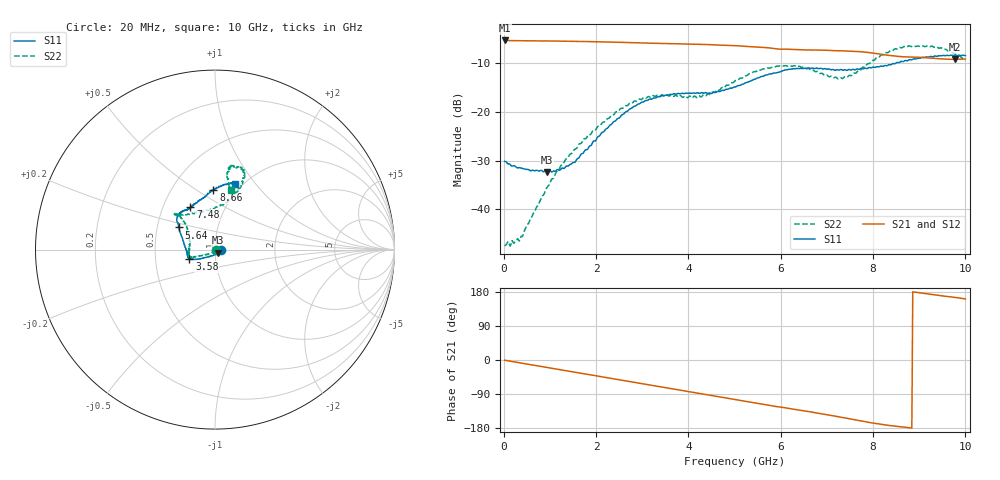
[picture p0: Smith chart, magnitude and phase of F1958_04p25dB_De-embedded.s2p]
! Integrated Device Technology
! Corporate Headquarters
! 6024 Silver Creek Valley Road
! San Jose, CA 95138  USA
! Phone:  1-408-284-8200
! Toll Free:  1-800-223-1366
! Webpage:  http://www.idt.com/
! Timing and RF Division
! 515 Groton Road, Suite 102
! Westford, MA 01886-6024
! Device:  F1958
! Description: 7-bit 0.25 dB Digital Step Attenuator
! Frequency:  0.001 -  6.000 GHz
! Package:  4x4 mm Thin QFN Plastic Package: 24 pin
! Ports:  2 RF, 12 DC
!  Pin  1  = D0
!  Pin  2  = VDD
!  Pin  3  = VMODE
!  Pin  4  = GND
!  Pin  5  = RF1  =  Port 1
!  Pin  6  = GND
!  Pin  7  = GND
!  Pin  8  = GND
!  Pin  9  = GND
!  Pin 10  = GND
!  Pin 11  = GND
!  Pin 12  = GND
!  Pin 13  = GND
!  Pin 14  = RF2  =  Port 2
!  Pin 15  = GND
!  Pin 16  = LE
!  Pin 17  = CLK
!  Pin 18  = DATA
!  Pin 19  = D6
!  Pin 20  = D5
!  Pin 21  = D4
!  Pin 22  = D3
!  Pin 23  = D2
!  Pin 24  = D1
! State:  17
! Atten State:  4.25 dB
! Voltage:  +3.30 Volts
! Current:  0.258 mA
! Data:  The device was measured on a F1958 evaluation board which has
!  individual transmission lines to the RF pins.  Data was collected
!  using a calibrated network analyzer.  The evaluation board was
!  de-embedded using Automatic Fixture Removal (AFR).
!  The reference plane is the edge of the package pin.
! Misc:
!  Action Tracker AT0419
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# GHz S dB R 50
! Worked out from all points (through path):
!   500 points, 20 MHz to 10 GHz, reference 50 ohm
!   highest |S21| = -5.27 dB at 20 MHz (marker M1); lowest = -9.2 dB at 9.78 GHz (marker M2)
!   group delay of S21, straight-line fit = 56.3 ps
!   lowest |S11| = -32.3 dB at 940 MHz (marker M3), VSWR 1.05, Z = 51.7 - j1.79 ohm
!   |S11| at or under -10 dB: start of sweep to 8.484 GHz
!   |S22| runs from -47.5 to -6.3 dB; largest |S21 - S12| = 0.0014
!   S11 on the Smith chart (normalised r, x): 20 MHz: 1.06, -0.00; 3.58 GHz: 0.75, -0.08; 5.64 GHz: 0.65, +0.17; 7.48 GHz: 0.69, +0.35; 8.66 GHz: 0.79, +0.59; 10 GHz: 0.93, +0.79
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0.02  -30.10 -3.8  -5.27 -0.6  -5.27 -0.5  -47.42 -25.6
0.38  -31.50 -13.7  -5.33 -8.1  -5.33 -8.1  -45.47 -90.0
0.94  -32.31 -45.4  -5.38 -19.8  -5.37 -19.8  -35.45 -122.3
1.34  -31.23 -85.8  -5.43 -28.2  -5.42 -28.2  -29.73 -138.7
1.7  -28.53 -112.3  -5.49 -35.6  -5.48 -35.6  -26.10 -148.8
2.58  -20.48 -146.7  -5.67 -54.0  -5.66 -54.0  -19.20 -159.2
2.94  -18.30 -153.2  -5.76 -61.4  -5.75 -61.5  -17.30 -161.2
3.36  -16.83 -157.7  -5.88 -70.1  -5.88 -70.2  -16.65 -164.5
3.58  -16.42 -160.3  -5.92 -74.6  -5.93 -74.7  -16.72 -168.9
4.32  -16.10 -171.9  -6.09 -89.9  -6.10 -90.0  -16.48 164.2
5.02  -14.83 165.7  -6.34 -104.7  -6.35 -104.7  -13.51 140.6
5.64  -12.55 148.4  -6.71 -117.6  -6.72 -117.6  -11.12 137.1
6.16  -11.24 140.7  -7.07 -127.4  -7.08 -127.4  -10.54 138.3
6.68  -10.95 133.2  -7.23 -137.6  -7.25 -137.5  -11.32 133.4
7.2  -11.33 125.0  -7.37 -148.6  -7.39 -148.4  -12.85 109.5
7.48  -11.23 120.0  -7.46 -154.7  -7.46 -154.6  -12.45 89.0
7.94  -10.88 109.3  -7.80 -165.2  -7.80 -165.2  -9.86 70.1
8.34  -10.26 99.2  -8.34 -172.6  -8.34 -172.7  -7.65 67.4
8.66  -9.61 91.6  -8.63 -177.0  -8.63 -177.0  -6.57 69.6
9.3  -8.61 78.6  -8.93 172.2  -8.93 172.2  -6.53 79.9
9.78  -8.28 74.1  -9.16 165.1  -9.18 165.1  -7.93 79.4
10  -8.39 73.0  -9.09 161.1  -9.12 161.2  -9.31 74.9
